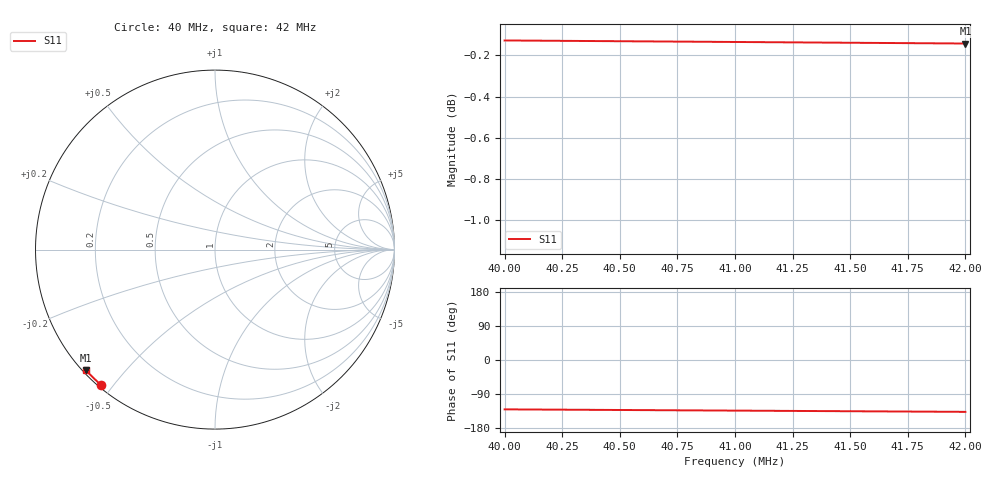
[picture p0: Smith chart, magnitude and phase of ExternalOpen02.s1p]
# Hz S RI R 50
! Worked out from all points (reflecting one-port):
!   9 points, 40 MHz to 42 MHz, reference 50 ohm
!   lowest |S11| = -0.1 dB at 42 MHz (marker M1), VSWR 122.11, Z = 0.473 - j19.8 ohm
!   phase of S11 starts at -130 deg and turns -7 deg over the sweep
4e7  -0.6369 -0.7519
4.025e7  -0.6475 -0.7426
4.05e7  -0.658 -0.733
4.075e7  -0.6683 -0.7234
4.1e7  -0.6785 -0.7135
4.125e7  -0.6885 -0.7036
4.15e7  -0.6984 -0.6935
4.175e7  -0.7081 -0.6832
4.2e7  -0.7177 -0.6728
